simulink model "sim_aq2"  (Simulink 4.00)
settings: Solver=ode45  StartTime=0.0  StopTime=10.0  RelTol=1e-3

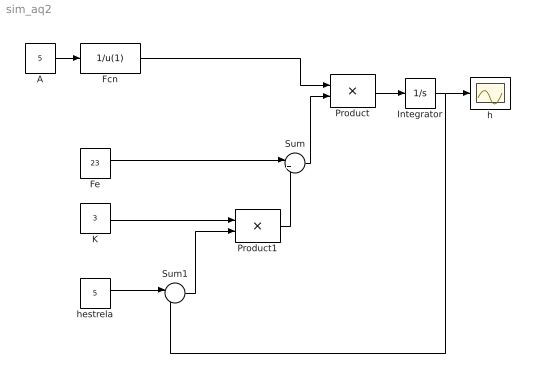
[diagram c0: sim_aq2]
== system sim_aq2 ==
  A : Constant  Value=5
  Fcn : Fcn  Expr=1/u(1)
  Fe : Constant  Value=23
  Integrator : Integrator  ExternalReset=none  InitialConditionSource=internal  InitialCondition=0  LimitOutput=off  UpperSaturationLimit=inf  LowerSaturationLimit=-inf  ShowSaturationPort=off  ShowStatePort=off  AbsoluteTolerance=auto
  K : Constant  Value=3
  Product : Product  Inputs=2  Multiplication=Element-wise(.*)  SaturateOnIntegerOverflow=on
  Product1 : Product  Inputs=2  Multiplication=Element-wise(.*)  SaturateOnIntegerOverflow=on
  Sum : Sum  Inputs=|+-  SaturateOnIntegerOverflow=on
  Sum1 : Sum  Inputs=|-+  SaturateOnIntegerOverflow=on
  h : Scope
  hestrela : Constant  Value=5
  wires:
  A/1 -> Fcn/1
  Fcn/1 -> Product/1
  Product/1 -> Integrator/1
  Integrator/1 -> h/1, Sum1/2
  Fe/1 -> Sum/1
  Sum/1 -> Product/2
  K/1 -> Product1/1
  Product1/1 -> Sum/2
  hestrela/1 -> Sum1/1
  Sum1/1 -> Product1/2
